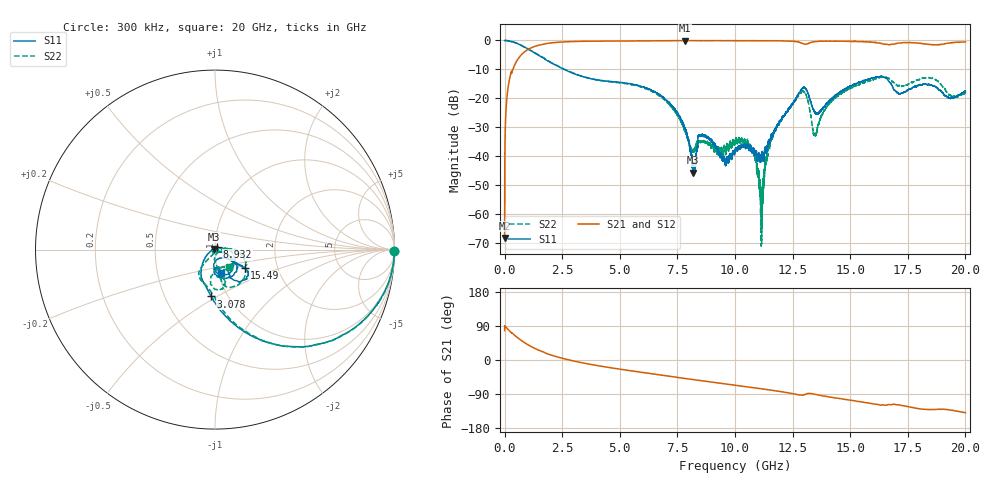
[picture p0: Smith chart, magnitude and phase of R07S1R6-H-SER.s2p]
!{R07S1R6}
!Johanson Technology Inc.
!www.johansontechnology.com
!Test Board Conditions:
!Substrate Type  RO4350B
!Substrate Thickness  10 mil
!Substrate Dk  3.66
!TL Type: GCPW
!TL Trace Width  21 mil
!TL Gap  20 mil
!Electrode orientation  Horizontal
!DUT TOPOLOGY	SERIES
!Mounting Pad LxW  16x21 mil
! Created Sat Feb  6 11:20:47 2021
# hz S ma R 50
! 2 Port Network Data from SP1.SP block
! freq  magS11  angS11  magS21  angS21  magS12  angS12  magS22  angS22
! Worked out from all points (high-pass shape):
!   20001 points, 300 kHz to 20 GHz, reference 50 ohm
!   highest |S21| = -0.05 dB at 7.838 GHz (marker M1); lowest = -68.3 dB at 300 kHz (marker M2)
!   |S21| within 3 dB of the highest: 1.032 GHz to end of sweep
!   lowest |S11| = -45.8 dB at 8.183 GHz (marker M3), VSWR 1.01, Z = 49.6 + j0.346 ohm
!   |S11| at or under -10 dB: 2.582 GHz to end of sweep
!   |S22| runs from -71.2 to 0.0 dB; largest |S21 - S12| = 0.012
!   S11 on the Smith chart (normalised r, x): 300 kHz: open; 3.078 GHz: 0.84, -0.47; 8.932 GHz: 1.02, +0.03; 15.49 GHz: 1.36, -0.29; 20 GHz: 1.03, -0.27
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300000  0.9987 -0.5  0.0003852 77.7  0.0003416 99.5  1 -0.6
1.313e8  0.99 -8.5  0.1343 81.7  0.1342 81.8  0.9906 -8.5
4.763e8  0.9096 -26.5  0.4064 63.2  0.4062 63.1  0.9119 -26.5
1.5843e9  0.5246 -66.9  0.8444 23.4  0.8465 23.4  0.5292 -65.7
3.0783e9  0.2617 -94.7  0.9604 -3.7  0.9614 -3.7  0.2637 -91.1
3.3343e9  0.2407 -97.9  0.9664 -6.9  0.9663 -7.0  0.2433 -94.2
6.6673e9  0.1197 -128.4  0.9887 -38.7  0.9884 -38.8  0.1144 -127.9
7.8383e9  0.02947 -158.1  0.9947 -48.8  0.9928 -48.8  0.02716 -110.6
8.1833e9  0.005153 137.5  0.9921 -51.7  0.9923 -51.7  0.01195 -45.3
8.4873e9  0.0226 46.4  0.9922 -54.2  0.9923 -54.3  0.01727 11.2
8.9323e9  0.01904 52.2  0.9905 -57.8  0.9905 -57.8  0.01579 -5.9
9.5243e9  0.01004 114.7  0.9911 -62.6  0.992 -62.7  0.01343 -82.8
1.00003e10  0.01271 179.9  0.9919 -66.6  0.9921 -66.7  0.01679 -125.4
1.07493e10  0.01185 -143.0  0.9882 -72.8  0.9896 -72.8  0.01243 -145.9
1.11533e10  0.0107 -89.1  0.9875 -76.0  0.9875 -76.2  0.001097 27.5
1.14963e10  0.01728 -34.9  0.9887 -79.1  0.9888 -79.1  0.01451 22.4
1.20033e10  0.04157 -18.4  0.9853 -83.6  0.9836 -83.6  0.04187 13.5
1.29563e10  0.1538 -55.2  0.8818 -92.3  0.8795 -92.4  0.1335 -45.3
1.33343e10  0.07476 -92.7  0.9327 -88.9  0.9329 -88.9  0.03871 -86.7
1.54913e10  0.1949 -32.4  0.9582 -110.6  0.9542 -110.6  0.1825 -20.1
1.66673e10  0.1991 -58.5  0.8411 -117.8  0.843 -118.2  0.2213 -70.6
2e10  0.1315 -75.5  0.9447 -139.0  0.9402 -139.0  0.1267 -51.4
